|Texas Instruments Incorporated
|Octal, Low Power, 12-Bit, +/-16.5 V Output Parallel Input Digital-To-Analog
|Converter
| Marketing part#   Digital Voltage Range   Package-type   #pins
| DAC7728SPAG   1.7V to 5.5V   TQFP   64
| DAC7728SPAGR   1.7V to 5.5V   TQFP   64
| DAC7728SRTQR   1.7V to 5.5V   QFN   56
| DAC7728SRTQT   1.7V to 5.5V   QFN   56
[IBIS Ver]   3.2
[File name]   dac7728.ibs
|SIMDE Ver   V2.2 - 201009 - RHL4 - Build 424
[File Rev]   1.0
[Date]   02/25/2011
[Source]
| Texas Instruments Incorporated.
| Analog-eLab Design Center, HPA
| 12500 TI Blvd
| Dallas, TX -75243
| e-mail: elab_ibis@list.ti.com
[Notes]   Revision History:
| Rev 1.0: 02/25/2011
| - Initial version of the model
| - Model generated from simulations in TISPICE
| - Model matched to SPICE simulation
| - C_comp although listed in numerical order of value are
|   obtained from varying PVT conditions. For PVT conditions for
|   each specific value refer the buffer description under
|   respective [Model]. IBIS model user is responsible for using
|   appropriate C_comp to simulate for Signal Integrity.
| - Model names with a trailing _1p8 contains the model for
|   1.8V [1.71V and 1.89V].Model names with a trailing _3p3 contains
|   the model for 3.3V [3.0V and 3.6V]. Model names with trailing _5
|   contains the model for 5.0V [4.5V and 5.5V] operation.
| - Rleative of DAC8728
[Disclaimer]
| This model is designed as an aid for customers of Texas Instruments.
| TI and its licensors and suppliers make no warranties, either expressed
| or implied, with respect to this  model, including the warranties of
| merchantability or fitness for a particular purpose. The model is
| provided solely on an "as is" basis. The entire risk as to its quality
| and performance is with the customer.
[Copyright]
 (C) Copyright 2011 Texas Instruments Incorporated.All rights reserved.
|   DAC7728RTQ
[Component]   DAC7728RTQ
[Manufacturer]   TI
[Package]   |56 QFN   -  RTQ package
|   typ   min   max
R_pkg   0.00127   0.00125   0.00140
L_pkg   0.18101nH   0.17521nH   0.20504nH
C_pkg   0.11787pF   0.10269pF   0.12129pF
[Pin]  signal_name   model_name   R_pin   L_pin   C_pin
1   D9   DATA   0.00137   0.20247nH  0.10293pF
2   D10   DATA   0.00125   0.17772nH  0.12127pF
3   D11   DATA   0.00125   0.17577nH  0.12129pF
4   VMON   TERM   0.00125   0.17533nH  0.12128pF
5   VOUT-3   TERM   0.00125   0.17523nH  0.12126pF
6   REF-A   TERM   0.00125   0.17521nH  0.12125pF
7   VOUT-2   TERM   0.00125   0.17521nH  0.12124pF
8   AVDD   POWER   0.00125   0.17523nH  0.12122pF
9   AGND-A   GND   0.00125   0.17527nH  0.12121pF
10   VOUT-1   TERM   0.00125   0.17535nH  0.12114pF
11   AVSS   POWER   0.00125   0.17551nH  0.12112pF
12   OFFSET-A   TERM   0.00125   0.17593nH  0.12114pF
13   VOUT-0   TERM   0.00125   0.17788nH  0.12117pF
14   _USB/BTCC   USB_RST   0.00139   0.20446nH  0.10371pF
15   _BUSY   BUSY   0.00138   0.20291nH  0.10270pF
16   _CLR   INPUT   0.00125   0.17796nH  0.12105pF
17   _LDAC   INPUT   0.00125   0.17600nH  0.12109pF
18   _RST   INPUT   0.00125   0.17554nH  0.12110pF
19   A0   INPUT   0.00125   0.17541nH  0.12111pF
20   A1   INPUT   0.00125   0.17537nH  0.12111pF
21   DVDD   POWER   0.00125   0.17535nH  0.12111pF
22   DGND   GND   0.00125   0.17535nH  0.12112pF
23   A2   INPUT   0.00125   0.17537nH  0.12111pF
24   A3   INPUT   0.00125   0.17544nH  0.12107pF
25   A4   INPUT   0.00125   0.17555nH  0.12108pF
26   DGND   GND   0.00125   0.17597nH  0.12111pF
27   GPIO   GPIO   0.00125   0.17791nH  0.12115pF
28   RSTSEL   USB_RST   0.00139   0.20448nH  0.10370pF
29   VOUT-7   TERM   0.00138   0.20291nH  0.10270pF
30   OFFSET-B   TERM   0.00125   0.17796nH  0.12105pF
31   AVSS   POWER   0.00125   0.17599nH  0.12109pF
32   VOUT-6   TERM   0.00125   0.17554nH  0.12110pF
33   AGND-B   GND   0.00125   0.17541nH  0.12111pF
34   AVDD   POWER   0.00125   0.17537nH  0.12111pF
35   VOUT-5   TERM   0.00125   0.17535nH  0.12111pF
36   REF-B   TERM   0.00125   0.17534nH  0.12113pF
37   VOUT-4   TERM   0.00125   0.17536nH  0.12113pF
38   NC   NC   0.00125   0.17541nH  0.12112pF
39   NC   NC   0.00125   0.17557nH  0.12106pF
40   NC   NC   0.00125   0.17601nH  0.12105pF
41   NC   NC   0.00125   0.17790nH  0.12115pF
42   NC   NC   0.00139   0.20448nH  0.10370pF
43   D0   DATA   0.00138   0.20293nH  0.10269pF
44   D1   DATA   0.00125   0.17800nH  0.12102pF
45   D2   DATA   0.00125   0.17605nH  0.12104pF
46   DGND   GND   0.00125   0.17563nH  0.12103pF
47   IOVDD   POWER   0.00125   0.17552nH  0.12101pF
48   DVDD   POWER   0.00125   0.17551nH  0.12099pF
49   R/_W   INPUT   0.00125   0.17550nH  0.12099pF
50   _CS   INPUT   0.00125   0.17556nH  0.12095pF
51   D3   DATA   0.00125   0.17557nH  0.12094pF
52   D4   DATA   0.00125   0.17565nH  0.12091pF
53   D5   DATA   0.00125   0.17579nH  0.12089pF
54   D6   DATA   0.00125   0.17625nH  0.12086pF
55   D7   DATA   0.00125   0.17825nH  0.12086pF
56   D8   DATA   0.00140   0.20504nH  0.10342pF
|   DAC7728PAG
[Component]   DAC7728PAG
[Manufacturer]   TI
[Package]   |64 TQFP  -  PAG package
|   typ   min   max
R_pkg   0.09996   0.05701   0.10904
L_pkg   3.35156nH   3.03842nH   3.68738nH
C_pkg   0.50033pF   0.43598pF   0.54508pF
[Pin]  signal_name   model_name   R_pin   L_pin   C_pin
1   D9   DATA   0.10566   3.62723nH  0.46020pF
2   D10   DATA   0.10159   3.45743nH  0.53671pF
3   D11   DATA   0.10000   3.35720nH  0.52701pF
4   VMON   TERM   0.10176   3.34678nH  0.50918pF
5   VOUT-3   TERM   0.10148   3.31393nH  0.50571pF
6   REF-A   TERM   0.10162   3.25664nH  0.48357pF
7   VOUT-2   TERM   0.10253   3.21700nH  0.47296pF
8   AVDD   POWER   0.05640   2.85004nH  0.48401pF
9   AGND-A   GND   0.05640   2.88385nH  0.48599pF
10   VOUT-1   TERM   0.10476   3.25937nH  0.48540pF
11   AVSS   POWER   0.05793   3.01181nH  0.53297pF
12   OFFSET-A   TERM   0.05701   3.03907nH  0.54508pF
13   VOUT-0   TERM   0.10486   3.40621nH  0.51117pF
14   NC   NC   0.00952   1.99807nH  0.43931pF
15   _USB/BTCC   USB_RST   0.09971   3.42490nH  0.52978pF
16   _BUSY   BUSY   0.10261   3.57554nH  0.45689pF
17   _CLR   INPUT   0.10804   3.67674nH  0.46169pF
18   _LDAC   INPUT   0.10384   3.50383nH  0.53542pF
19   _RST   INPUT   0.10820   3.51169nH  0.53466pF
20   A0   INPUT   0.10606   3.43047nH  0.51577pF
21   A1   INPUT   0.10458   3.37513nH  0.50308pF
22   NC   NC   0.00916   1.86104nH  0.39171pF
23   NC   NC   0.00889   1.80020nH  0.38069pF
24   DVDD   POWER   0.05377   2.70150nH  0.47681pF
25   DGND   GND   0.05395   2.69082nH  0.48509pF
26   A2   INPUT   0.09806   3.14045nH  0.46810pF
27   A3   INPUT   0.09732   3.18322nH  0.47406pF
28   NC   NC   0.00943   1.92658nH  0.41197pF
29   A4   INPUT   0.09635   3.25388nH  0.49904pF
30   DGND   GND   0.09406   3.25402nH  0.51527pF
31   NC   NC   0.00979   2.07445nH  0.44475pF
32   NC   NC   0.00986   2.17258nH  0.36899pF
33   GPIO   GPIO   0.10262   3.57573nH  0.45600pF
34   RSTSEL   USB_RST   0.09972   3.42583nH  0.52906pF
35   NC   NC   0.00952   1.99850nH  0.43874pF
36   VOUT-7   TERM   0.10486   3.40638nH  0.51087pF
37   OFFSET-B   TERM   0.05701   3.03842nH  0.54504pF
38   AVSS   POWER   0.05792   3.01056nH  0.53313pF
39   VOUT-6   TERM   0.10476   3.25940nH  0.48545pF
40   AGND-B   GND   0.05640   2.88225nH  0.48609pF
41   AVDD   POWER   0.05640   2.85149nH  0.48388pF
42   VOUT-5   TERM   0.10253   3.21717nH  0.47285pF
43   REF-B   TERM   0.10163   3.25742nH  0.48288pF
44   VOUT-4   TERM   0.10149   3.31419nH  0.50108pF
45   NC   NC   0.00937   1.95351nH  0.41976pF
46   NC   NC   0.10000   3.35687nH  0.52714pF
47   NC   NC   0.10262   3.47520nH  0.53964pF
48   NC   NC   0.10716   3.65444nH  0.46174pF
49   NC   NC   0.10605   3.63275nH  0.45770pF
50   D0   DATA   0.10554   3.52693nH  0.53845pF
51   D1   DATA   0.10218   3.39359nH  0.53245pF
52   D2   DATA   0.09950   3.30245nH  0.50826pF
53   NC   NC   0.00943   1.92643nH  0.41193pF
54   DGND   GND   0.05428   2.78415nH  0.52691pF
55   IOVDD   POWER   0.09831   3.13580nH  0.47407pF
56   DVDD   POWER   0.05443   2.69518nH  0.48680pF
57   R/_W   INPUT   0.09969   3.15690nH  0.43598pF
58   _CS   INPUT   0.09829   3.13555nH  0.47210pF
59   D3   DATA   0.09855   3.19662nH  0.48223pF
60   D4   DATA   0.09979   3.27938nH  0.50309pF
61   D5   DATA   0.10124   3.33408nH  0.51014pF
62   D6   DATA   0.10041   3.36062nH  0.52890pF
63   D7   DATA   0.10336   3.48625nH  0.53916pF
64   D8   DATA   0.10904   3.68738nH  0.46353pF
|   Model Selectors
[Model Selector] INPUT
input_1p8  1.8V digital input
input_3p3  3.3V digital input
input_5   5.0V digital input
[Model Selector] USB_RST
usb_rst_1p8   1.8V digital input
usb_rst_3p3   3.3V digital input
usb_rst_5   5.0V digital input
[Model Selector] DATA
data_1p8   1.8V digital I/O
data_3p3   3.3V digital I/O
data_5   5.0V digital I/O
[Model Selector] GPIO
gpio_1p8   1.8V digital I/O_open_drain
gpio_3p3   3.3V digital I/O_open_drain
gpio_5   5.0V digital I/O_open_drain
[Model Selector] BUSY
busy_1p8   1.8V digital Open_drain
busy_3p3   3.3V digital Open_drain
busy_5   5.0V digital Open_drain
[Model Selector] TERM
term_1-8V  1.8V nominal termination
term_3-3V  3.3V nominal termination
term_5-0V  5.0V nominal termination
[Model]  term_1-8V
Model_type Terminator
C_comp   1.0e-20F  1.0e-20F  1.0e-20F
|   typ   min   max
[Voltage Range]   1.8V   1.71V   1.89V
[POWER Clamp Reference]   1.8V   1.71V   1.89V
[GND Clamp Reference]   0V   0V   0V
|Ambient Temperature   25   105   -40
|Junction Temperature
[Temperature Range]   33   113   -40
[Model]  term_3-3V
Model_type Terminator
C_comp   1.0e-20F  1.0e-20F  1.0e-20F
|   typ   min   max
[Voltage Range]   3.3V   3.0V   3.6V
[POWER Clamp Reference]   3.3V   3.0V   3.6V
[GND Clamp Reference]   0V   0V   0V
|Ambient Temperature   25   105   -40
|Junction Temperature
[Temperature Range]   33   113   -40
[Model]  term_5-0V
Model_type Terminator
C_comp   1.0e-20F  1.0e-20F  1.0e-20F
|   typ   min   max
[Voltage Range]   5.0V   4.5V   5.5V
[POWER Clamp Reference]   5.0V   4.5V   5.5V
[GND Clamp Reference]   0V   0V   0V
|Ambient Temperature   25   105   -40
|Junction Temperature
[Temperature Range]   33   113   -40
| Models and submodels in the file (18): input_1p8 (Input), input_3p3 (Input), input_5 (Input), usb_rst_1p8 (Input), usb_rst_3p3 (Input), usb_rst_5 (Input), data_1p8 (I/O), data_3p3 (I/O), data_5 (I/O), gpio_1p8 (I/O_open_drain), gpio_3p3 (I/O_open_drain), gpio_5 (I/O_open_drain), busy_1p8 (Open_drain), busy_3p3 (Open_drain), busy_5 (Open_drain), term_1-8V (Terminator), term_3-3V (Terminator), term_5-0V (Terminator)
